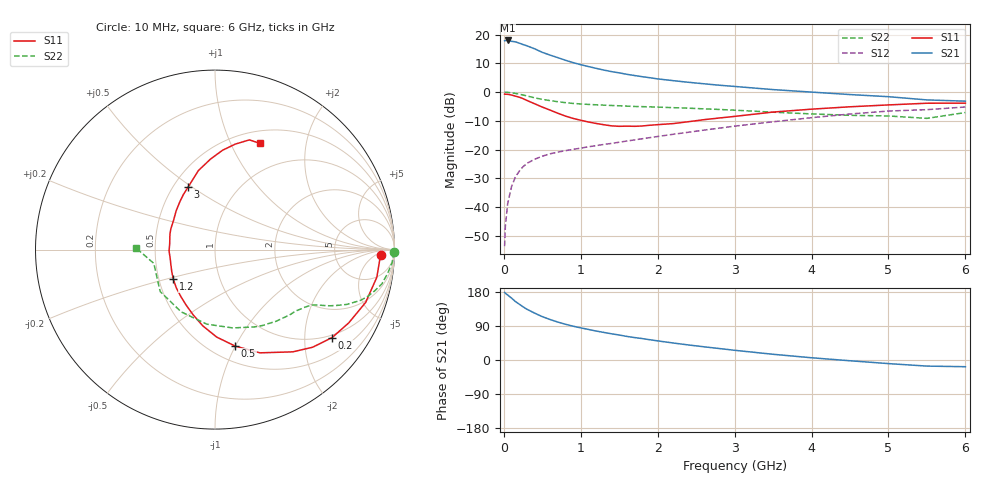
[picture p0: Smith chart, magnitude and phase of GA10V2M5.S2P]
! Infineon Technologies  Discrete & RF Semiconductors
! BF775
! Si NPN RF Bipolar Junction Transistor in SOT23
! VCE = 10 V  IC = 2.5 mA
! Common Emitter S-Parameters:  May  1996
# GHz  S  MA  R  50
!  f  S11  S21  S12  S22
! GHz  MAG  ANG  MAG  ANG  MAG  ANG  MAG  ANG
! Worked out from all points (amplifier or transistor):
!   36 points, 10 MHz to 6 GHz, reference 50 ohm
!   highest |S21| = 17.9 dB at 50 MHz (marker M1)
!   |S21| within 3 dB of that: start of sweep to 407.9 MHz
!   unconditionally stable (mu >= 1): 1.144 GHz to 3.125 GHz
!   at 250 MHz: K = 0.32, MSG = 21.2 dB, |S12| = -25.9 dB
!   at 1.4 GHz: K = 1.09, MAG = 10.7 dB, |S12| = -17.8 dB
!   at 6 GHz: K = 0.91, MSG = 1.0 dB, |S12| = -5.2 dB
!   S11 on the Smith chart (normalised r, x): 10 MHz: 21, -9; 200 MHz: 0.93, -2.72; 500 MHz: 0.65, -1.00; 1.2 GHz: 0.59, -0.21; 3 GHz: 0.59, +0.48; 6 GHz: 0.64, +1.30
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0.01  0.9228 -1.9  7.788 178.3  0.0021 85.3  0.9976 -0.8
0.02  0.9188 -4.1  7.887 176.2  0.0047 85.3  0.9944 -1.6
0.05  0.9147 -9.7  7.897 171.4  0.0116 85.2  0.9901 -4.1
0.1  0.8895 -19.3  7.62 163.4  0.0227 79.0  0.9709 -7.9
0.15  0.8498 -28.7  7.482 154.3  0.0334 73.6  0.9492 -11.6
0.2  0.816 -36.9  7.102 147.4  0.0422 69.8  0.9187 -14.5
0.3  0.7161 -52.7  6.377 133.9  0.0577 62.6  0.8574 -19.3
0.4  0.6272 -66.5  5.654 123.7  0.0681 57.5  0.7952 -22.6
0.5  0.549 -78.2  4.905 114.4  0.0768 54.7  0.747 -24.6
0.6  0.4874 -88.9  4.402 106.9  0.0846 52.3  0.7116 -26.1
0.7  0.4302 -99.1  3.977 100.2  0.0904 51.4  0.6815 -27.2
0.8  0.3834 -108.5  3.578 94.4  0.0959 50.6  0.6558 -28.1
0.9  0.3488 -117.4  3.256 89.2  0.1011 50.6  0.6354 -29.0
1.1  0.3024 -135.7  2.778 80.6  0.1121 51.1  0.6107 -30.9
1.2  0.2851 -144.6  2.587 76.4  0.1174 51.2  0.601 -31.9
1.6  0.2562 -178.4  2.038 62.2  0.1412 52.9  0.5702 -36.4
2.2  0.2834 144.3  1.581 44.9  0.1847 54.0  0.5362 -45.5
3  0.3782 113.5  1.254 25.6  0.2559 51.1  0.4848 -62.6
3.5  0.4498 101.9  1.105 15.1  0.305 47.1  0.4474 -77.3
4.5  0.5555 85.6  0.906 -2.0  0.416 36.0  0.3947 -118.6
5.5  0.6406 72.6  0.731 -16.1  0.4954 19.7  0.3494 -167.3
6  0.6426 67.0  0.696 -17.7  0.5509 15.2  0.4414 178.7
